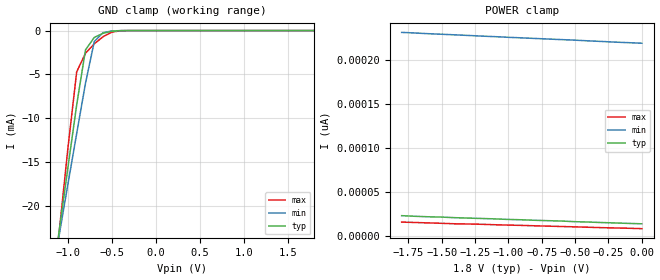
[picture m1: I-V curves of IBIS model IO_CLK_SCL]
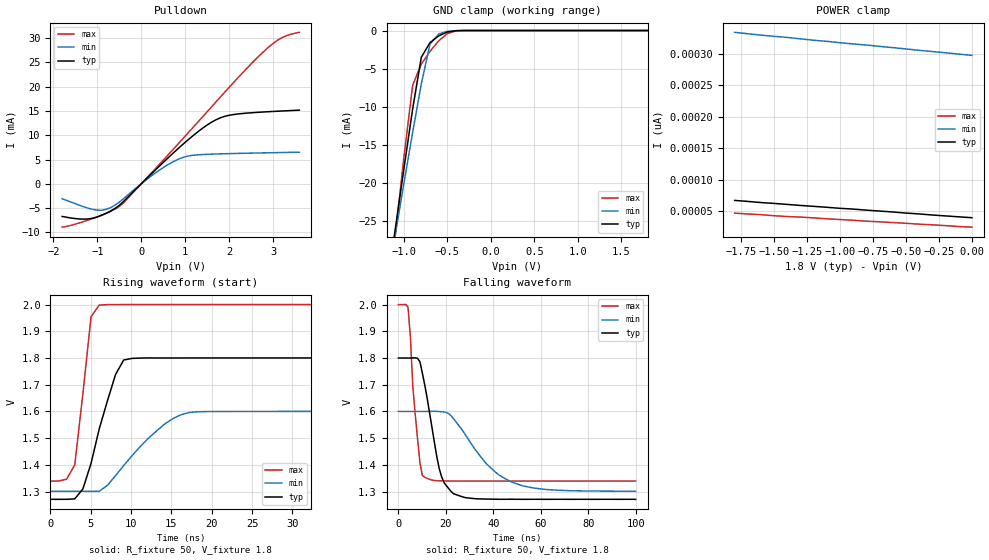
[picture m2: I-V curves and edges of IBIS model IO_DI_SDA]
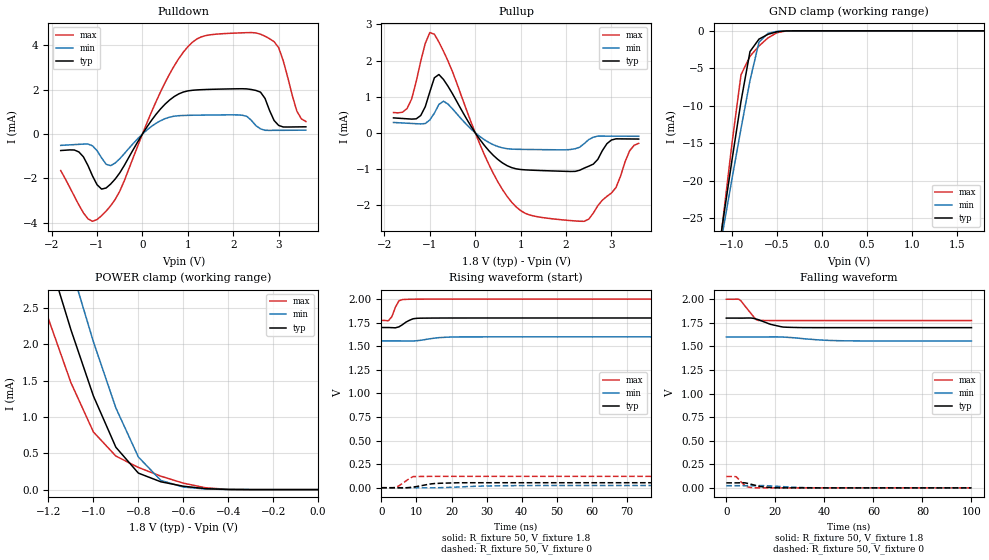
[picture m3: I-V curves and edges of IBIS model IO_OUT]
[IBIS Ver]   3.2
[Comment Char]   |_char
[File name]   rx6110sa_18v.ibs
[File Rev]   1.0
[Date]   2014/01/14 19:07:53
[Source]   This file orginated at SEIKO EPSON Corp.
[Copyright]
   Copyright 2013, SEIKO EPSON Corp.
[Component]   6110sa_18
[Manufacturer]   SEIKO EPSON Corp.
[Package]
| variable   typ   min   max
R_pkg   3.00m   NA   NA
L_pkg   3.70nH   NA   NA
C_pkg   0.70pF   NA   NA
[Pin] signal_name   model_name
1   CLK/SCL   IO_CLK_SCL
2   DI/SDA   IO_DI_SDA
3   DO/FOUT   IO_OUT
4   CE/FOE   IO_CE
5   SPISEL   IO_SPISEL
6   GND   GND
7   /IRQ2   IO_IRQ2
8   NC   NC
9   VBAT   POWER
10   VDD   POWER
11   VIO   POWER
12   /IRQ1   IO_NOD
13   NC   NC
14   NC   NC
| Models and submodels in the file (7): IO_CLK_SCL (Input), IO_DI_SDA (I/O_open_drain), IO_OUT (3-state), IO_CE (Input), IO_SPISEL (Input), IO_IRQ2 (3-state), IO_NOD (Open_drain)
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[Model]   IO_CLK_SCL
Model_type Input
Enable Active-Low
Polarity Non-Inverting
Vinh=1.26
Vinl=0.54
C_comp   2.5p   2p   3p
[Temperature Range] 25   85   -40
[Voltage Range]   1.8   1.6   2.0
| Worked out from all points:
|   GND clamp passes 1 mA (typ) near -0.72 V on its own axis
[GND Clamp]
-1.8V     -75.19mA   -65.43mA   -91.91mA
-1.1V     -22.89mA   -23.37mA   -23.06mA
-1V       -15.64mA   -17.52mA   -13.43mA
-900mV    -8.46mA    -11.72mA   -4.701mA
-800mV    -2.2mA     -5.996mA   -2.58mA
-700mV    -777.8uA   -1.246mA   -1.512mA
-600mV    -308.2uA   -237.4uA   -691.5uA
-500mV    -74.58uA   -42.13uA   -176.4uA
-400mV    -7.855uA   -4.907uA   -14.74uA
1.8V      13.7pA     219.9pA    7.39pA
[POWER Clamp]
-1.8V     22.96pA    230.9pA    15.69pA
-1.7V     22.28pA    230.2pA    15.23pA
-1.6V     21.71pA    229.4pA    14.78pA
-1.5V     21.37pA    228.8pA    14.32pA
-1.4V     20.69pA    228.1pA    13.76pA
-1.2V     19.78pA    226.7pA    13.19pA
-1.1V     19.33pA    226.1pA    12.68pA
-1V       18.7pA     225.3pA    12.28pA
-600mV    16.88pA    222.7pA    10.69pA
-500mV    16.14pA    222.1pA    10.29pA
-200mV    14.72pA    219.9pA    9.038pA
0V        13.76pA    218.6pA    8.242pA
[Model]   IO_DI_SDA
Model_type I/O_open_drain
Enable Active-Low
Polarity Non-Inverting
Vinh=1.26
Vinl=0.54
Vref=1.8
Vmeas=0.9
Rref=5000
C_comp   2.5p   2p   3p
[Temperature Range] 25   85   -40
[Voltage Range]   1.8   1.6   2.0
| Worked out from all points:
|   slope of the pulldown table from 0 to 0.27 V, typ, clamps not added: 113 ohm
|   GND clamp passes 1 mA (typ) near -0.63 V on its own axis
|   falling waveform, R_fixture 50, V_fixture 1.8: 20-80 % time 6.31ns typ, 16.5ns min, 3.25ns max; typ from 1.8 V to 1.27 V
|   rising waveform, R_fixture 50, V_fixture 1.8: 20-80 % time 2.89ns typ, 5.57ns min, 1.44ns max; typ from 1.27 V to 1.8 V
[Pulldown]
-1.8V     -6.712mA   -3.071mA   -8.913mA
-1.3V     -7.265mA   -4.749mA   -7.727mA
-1V       -6.813mA   -5.412mA   -6.785mA
-800mV    -6.068mA   -5.261mA   -6.079mA
-500mV    -4.43mA    -3.774mA   -4.657mA
300mV     2.653mA    2.091mA    2.898mA
800mV     6.924mA    4.885mA    7.817mA
1.4V      11.46mA    6.029mA    13.82mA
1.8V      13.58mA    6.164mA    17.84mA
3V        14.89mA    6.406mA    28.87mA
3.3V      15.03mA    6.458mA    30.46mA
3.6V      15.16mA    6.509mA    31.17mA
[GND Clamp]
-1.8V     -85.68mA   -77.18mA   -101.5mA
-1.1V     -26.07mA   -26.85mA   -26.94mA
-1V       -18.1mA    -20.02mA   -16.6mA
-900mV    -10.31mA   -13.38mA   -7.181mA
-800mV    -3.5mA     -6.992mA   -4.403mA
-700mV    -1.586mA   -1.78mA    -2.72mA
-600mV    -706.9uA   -462.6uA   -1.348mA
-500mV    -194.3uA   -99.1uA    -403.3uA
-400mV    -22.61uA   -12.12uA   -41.38uA
1.8V      39.62pA    301.7pA    22.28pA
[POWER Clamp]
-1.8V     67.19pA    334.1pA    46.95pA
-1.6V     63.78pA    329.7pA    44.57pA
-1.5V     62.41pA    327.8pA    42.86pA
-1.4V     60.82pA    326.1pA    41.61pA
-1.2V     57.75pA    321.6pA    39.45pA
-1.1V     56.27pA    319.8pA    38.03pA
-1V       54.63pA    317.6pA    36.83pA
-900mV    53.43pA    315.7pA    35.7pA
-800mV    51.73pA    313.9pA    34.22pA
-300mV    44pA       303.6pA    28.42pA
-100mV    41.15pA    299.6pA    25.75pA
0V        39.73pA    297.6pA    24.73pA
[Falling Waveform]
R_fixture=50
V_fixture=1.8
V_fixture_min=1.6
V_fixture_max=2.0
0s        1.8V       1.6V       2V
4.04ns    1.8V       1.6V       1.991V
6.061ns   1.8V       1.6V       1.696V
8.081ns   1.799V     1.6V       1.497V
9.091ns   1.786V     1.6V       1.407V
11.11ns   1.699V     1.6V       1.353V
17.17ns   1.388V     1.6V       1.34V
23.23ns   1.292V     1.573V     1.339V
47.47ns   1.271V     1.337V     1.339V
100ns     1.271V     1.301V     1.339V
[Rising Waveform]
R_fixture=50
V_fixture=1.8
V_fixture_min=1.6
V_fixture_max=2.0
0s        1.271V     1.301V     1.339V
2.02ns    1.271V     1.301V     1.346V
3.03ns    1.273V     1.301V     1.4V
5.051ns   1.405V     1.301V     1.955V
6.061ns   1.534V     1.301V     1.998V
8.081ns   1.738V     1.36V      2V
9.091ns   1.792V     1.397V     2V
14.14ns   1.8V       1.552V     2V
17.17ns   1.8V       1.596V     2V
100ns     1.8V       1.6V       2V
[Ramp]
R_load=50
dV/dt_r   3.174E-1/2.855E-9   1.793E-1/5.556E-9   3.964E-1/1.414E-9
dV/dt_f   3.174E-1/6.286E-9   1.792E-1/1.650E-8   3.964E-1/3.238E-9
|[End   IO_DI_SDA
[Model]   IO_OUT
Model_type 3-state
Enable Active-High
Polarity Non-Inverting
Vmeas=0.90
C_comp   2.5p   2p   3p
[Temperature Range] 25   85   -40
[Voltage Range]   1.8   1.6   2.0
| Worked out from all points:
|   slope of the pulldown table from 0 to 0.27 V, typ, clamps not added: 335 ohm
|   slope of the pullup table from 0 to 0.27 V, typ, clamps not added: 599 ohm
|   GND clamp passes 1 mA (typ) near -0.68 V on its own axis
|   POWER clamp passes 1 mA (typ) near -0.96 V on its own axis
|   falling waveform, R_fixture 50, V_fixture 1.8: 20-80 % time 7.15ns typ, NA min, 4.16ns max; typ from 1.8 V to 1.7 V
|   falling waveform, R_fixture 50, V_fixture 0: 20-80 % time 5.43ns typ, NA min, 2.83ns max; typ from 0.053 V to 0 V
|   rising waveform, R_fixture 50, V_fixture 1.8: 20-80 % time 2.69ns typ, NA min, 1.56ns max; typ from 1.7 V to 1.8 V
|   rising waveform, R_fixture 50, V_fixture 0: 20-80 % time 4.92ns typ, NA min, 2.81ns max; typ from 0 V to 0.053 V
[Pullup]
-1.8V     413.3uA    286.5uA    561.7uA
-1.5V     388.1uA    266uA      674.5uA
-1.2V     479.5uA    246.2uA    1.984mA
-1V       1.135mA    356.7uA    2.776mA
-900mV    1.524mA    543.7uA    2.731mA
-700mV    1.478mA    875.9uA    2.261mA
600mV     -833.9uA   -416.9uA   -1.572mA
1V        -1.016mA   -458.5uA   -2.155mA
1.6V      -1.052mA   -467.6uA   -2.367mA
2.5V      -924.6uA   -188.6uA   -2.391mA
3V        -199.5uA   -92.46uA   -1.668mA
3.6V      -172.6uA   -96.03uA   -292uA
[Pulldown]
-1.8V     -744.1uA   -511.6uA   -1.645mA
-1.2V     -1.419mA   -450uA     -3.823mA
-900mV    -2.482mA   -1.074mA   -3.68mA
-500mV    -1.752mA   -1.114mA   -2.578mA
700mV     1.689mA    804uA      3.073mA
1.4V      2.007mA    854.6uA    4.439mA
2.2V      2.041mA    847.2uA    4.561mA
2.6V      1.888mA    234uA      4.498mA
2.9V      608.2uA    165.3uA    4.161mA
3.1V      317.4uA    167.6uA    3.309mA
3.4V      320.6uA    171uA      1.036mA
3.6V      325.4uA    173.4uA    564.4uA
[GND Clamp]
-1.8V     -84.94mA   -76.24mA   -100.6mA
-1.2V     -33.65mA   -33.58mA   -35.52mA
-1.1V     -25.34mA   -26.62mA   -25.12mA
-1V       -17.22mA   -19.74mA   -14.99mA
-900mV    -9.404mA   -13.04mA   -5.869mA
-800mV    -2.766mA   -6.628mA   -3.399mA
-700mV    -1.108mA   -1.501mA   -2.022mA
-600mV    -467.2uA   -331.2uA   -944.2uA
-500mV    -123.2uA   -66.32uA   -251.8uA
-400mV    -14.38uA   -8.214uA   -22.27uA
1.8V      25.69pA    24.39nA    13.13pA
[POWER Clamp]
-1.8V     9.515mA    10.63mA    8.378mA
-1.3V     4.242mA    5.194mA    3.317mA
-1.2V     3.21mA     4.128mA    2.351mA
-1.1V     2.201mA    3.07mA     1.473mA
-1V       1.29mA     2.036mA    794.1uA
-900mV    583.1uA    1.124mA    461.8uA
-800mV    227.2uA    449.5uA    305.5uA
-700mV    107.6uA    126.8uA    185uA
-600mV    46.57uA    34.75uA    88.82uA
-500mV    12.68uA    8.521uA    25.07uA
-400mV    1.719uA    1.484uA    2.421uA
0V        25.86pA    267.4pA    16.26pA
[Falling Waveform]
R_fixture=50
V_fixture=1.8
V_fixture_min=1.6
V_fixture_max=2.0
0s        1.8V       1.6V       2V
5.051ns   1.8V       1.6V       2V
6.061ns   1.8V       1.6V       1.981V
10.1ns    1.801V     1.6V       1.848V
12.12ns   1.79V      1.6V       1.785V
13.13ns   1.783V     1.6V       1.775V
18.18ns   1.733V     1.601V     1.774V
24.24ns   1.704V     1.597V     1.774V
46.46ns   1.699V     1.56V      1.774V
100ns     1.699V     1.557V     1.774V
[Falling Waveform]
R_fixture=50
V_fixture=0
V_fixture_min=0
V_fixture_max=0
0s        52.88mV    23.36mV    120.3mV
4.04ns    52.83mV    23.37mV    118mV
6.061ns   54.11mV    23.36mV    60.91mV
8.081ns   50.96mV    23.35mV    16.4mV
10.1ns    38.07mV    23.4mV     3.78mV
12.12ns   24.5mV     23.8mV     238.5uV
15.15ns   9.607mV    23.98mV    99.72uV
21.21ns   297.5uV    15.58mV    4.292uV
37.37ns   2.958uV    511.9uV    0V
100ns     0V         -26.06uV   0V
[Rising Waveform]
R_fixture=50
V_fixture=1.8
V_fixture_min=1.6
V_fixture_max=2.0
0s        1.699V     1.557V     1.774V
2.02ns    1.699V     1.557V     1.77V
3.03ns    1.697V     1.557V     1.815V
4.04ns    1.696V     1.557V     1.916V
5.051ns   1.706V     1.557V     1.983V
7.071ns   1.757V     1.556V     1.998V
9.091ns   1.792V     1.556V     1.999V
12.12ns   1.798V     1.569V     2V
20.2ns    1.8V       1.599V     2V
100ns     1.8V       1.6V       2V
[Rising Waveform]
R_fixture=50
V_fixture=0
V_fixture_min=0
V_fixture_max=0
0s        0V         0V         0V
4.04ns    -73.17uV   936.3nV    3.023mV
5.051ns   -751.5uV   14.86uV    20.81mV
8.081ns   2.632mV    32.05uV    98.73mV
9.091ns   6.924mV    -116.7uV   118.2mV
15.15ns   44.25mV    -586.8uV   120.5mV
22.22ns   52.64mV    8.175mV    120.3mV
29.29ns   52.88mV    17.86mV    120.3mV
39.39ns   52.88mV    22.52mV    120.3mV
100ns     52.87mV    23.37mV    120.3mV
[Ramp]
R_load=50
dV/dt_r   3.172E-2/4.868E-9   1.402E-2/1.045E-8   7.219E-2/2.793E-9
dV/dt_f   6.070E-2/7.148E-9   2.574E-2/1.250E-8   1.357E-1/4.163E-9
|[End   IO_OUT
